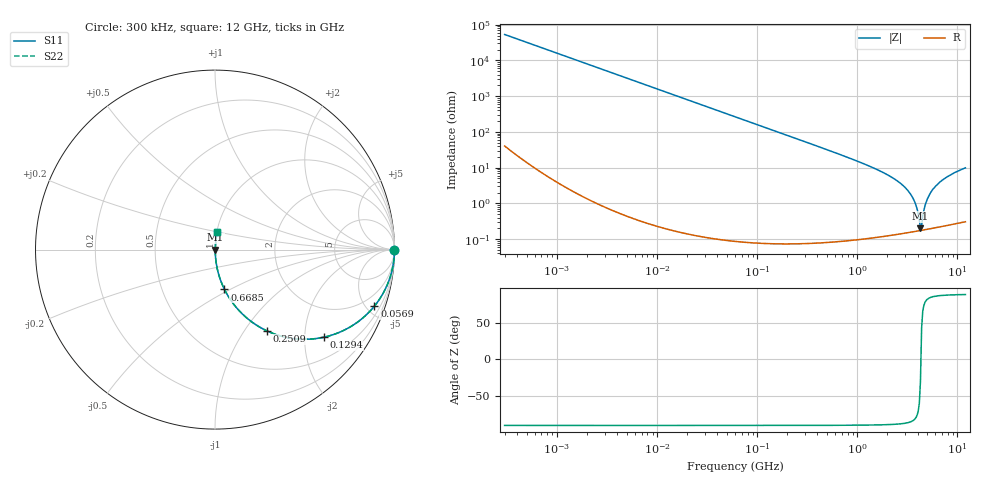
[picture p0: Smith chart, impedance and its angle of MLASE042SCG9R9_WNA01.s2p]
! MLASE042SCG9R9_WNA01  S-PARAMETER MODEL  ( General Type )
! Model Generated by TAIYO YUDEN Corporation (http://www.ty-top.com)
! Version 1.0
! TAIYO YUDEN Control No. 130801
! Copyright(c) 2013 TAIYO YUDEN CO.,LTD. All Rights Reserved.
! Product Description (link to TY-COMPAS)
! https://ds.yuden.co.jp/TYCOMPAS/or/detail?pn=MLASE042SCG9R9BWNA01&u=M
! Products Name : Multilayer Ceramic Capacitors
! Characteristics :
!  Capacitance : 9.9 pF , Rated Voltage : 16V , TCC : CG / C0G
!  Case Size : 0.4 x 0.2 / 0.016 x 0.008 [mm/inch] , Thickness : 0.2 / 0.008 [mm/inch]
!  (Conditions: Temperature = 25 degC , DC Bias Current/Voltage = 0A / 0V)
! External Node Assignments :
!  1  o---| |---o  2
! GND o---------o GND
! Frequency Range : 0.3MHz  -  12000MHz  [ 401 STEP ]
# MHz S RI R 50
! Freq[MHz].  S11 Real  S11 Imag  S21 Real  S21 Imag  S12 Real  S12 Imag  S22 Real  S22 Imag
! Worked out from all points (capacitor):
!   401 points, 300 kHz to 12 GHz, reference 50 ohm
!   read as one part in series: C = 9.91 pF near 316.3 kHz
!   lowest |Z| = 200 mohm at 4.271 GHz (marker M1)
!   series resonance near 4.314 GHz, so ESL is about 140 pH
!   S11 on the Smith chart (normalised r, x): 300 kHz: open; 56.9 MHz: 1.00, -5.64; 129.4 MHz: 1.00, -2.48; 250.9 MHz: 1.00, -1.28; 668.5 MHz: 1.00, -0.47; 12 GHz: 1.01, +0.20
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0.3  1 -0.00187  4.9e-06 0.00187  4.9e-06 0.00187  1 -0.00187
1.769972  0.9999 -0.011  0.000123 0.011  0.000123 0.011  0.9999 -0.011
10.44266  0.9958 -0.0648  0.00422 0.0648  0.00422 0.0648  0.9958 -0.0648
25.70316  0.975 -0.1561  0.025 0.1561  0.025 0.1561  0.975 -0.1561
56.90376  0.8883 -0.3149  0.1117 0.3149  0.1117 0.3149  0.8883 -0.3149
60  0.8773 -0.3279  0.1227 0.3279  0.1227 0.3279  0.8773 -0.3279
129.3602  0.6058 -0.4884  0.3942 0.4884  0.3942 0.4884  0.6058 -0.4884
250.8588  0.2894 -0.4529  0.7106 0.4529  0.7106 0.4529  0.2894 -0.4529
353.9943  0.1691 -0.374  0.8309 0.374  0.8309 0.374  0.1691 -0.374
668.5285  0.0528 -0.2218  0.9472 0.2218  0.9472 0.2218  0.0528 -0.2218
2088.533  0.0047 -0.0586  0.9953 0.0586  0.9953 0.0586  0.0047 -0.0586
2795.104  0.00253 -0.0334  0.9975 0.0334  0.9975 0.0334  0.00253 -0.0334
3364.605  0.0019 -0.0188  0.9981 0.0188  0.9981 0.0188  0.0019 -0.0188
3740.715  0.00174 -0.0108  0.9983 0.0108  0.9983 0.0108  0.00174 -0.0108
4158.869  0.00172 -0.00297  0.9983 0.00297  0.9983 0.00297  0.00172 -0.00297
4270.516  0.00174 -0.000983  0.9983 0.000983  0.9983 0.000983  0.00174 -0.000983
4502.883  0.0018 0.00401  0.9982 -0.00401  0.9982 -0.00401  0.0018 0.00401
4747.894  0.0019 0.00854  0.9981 -0.00854  0.9981 -0.00854  0.0019 0.00854
5006.236  0.00205 0.0131  0.9979 -0.0131  0.9979 -0.0131  0.00205 0.0131
5868.704  0.00278 0.0271  0.9972 -0.0271  0.9972 -0.0271  0.00278 0.0271
7854.144  0.00537 0.0544  0.9946 -0.0544  0.9946 -0.0544  0.00537 0.0544
12000  0.0126 0.0972  0.9874 -0.0972  0.9874 -0.0972  0.0126 0.0972
